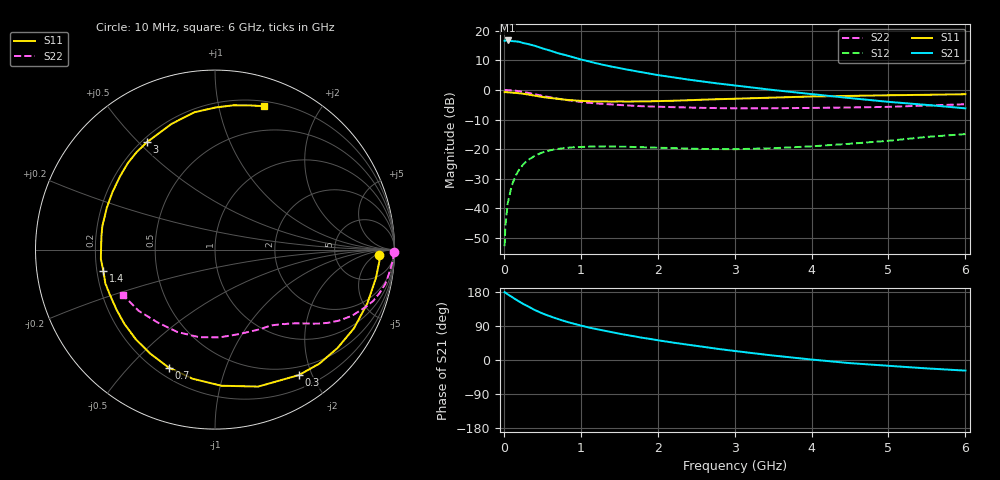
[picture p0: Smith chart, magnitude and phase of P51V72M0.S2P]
! SIEMENS Small Signal Semiconductors
! BFP183
! Si NPN RF Bipolar Junction Transistor in SOT143
! VCE = 1.75 V  IC = 2 mA
! Common Emitter S-Parameters:  March  1996
# GHz  S  MA  R  50
!  f  S11  S21  S12  S22
! GHz  MAG  ANG  MAG  ANG  MAG  ANG  MAG  ANG
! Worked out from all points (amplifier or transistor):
!   36 points, 10 MHz to 6 GHz, reference 50 ohm
!   highest |S21| = 16.7 dB at 50 MHz (marker M1)
!   |S21| within 3 dB of that: start of sweep to 545.6 MHz
!   unconditionally stable (mu >= 1): 2.063 GHz to end of sweep
!   at 250 MHz: K = 0.12, MSG = 20.5 dB, |S12| = -25.2 dB
!   at 1.4 GHz: K = 0.68, MSG = 13.5 dB, |S12| = -19.1 dB
!   at 6 GHz: K = 1.01, MAG = 3.8 dB, |S12| = -14.9 dB
!   S11 on the Smith chart (normalised r, x): 10 MHz: 20, -7; 300 MHz: 0.38, -1.81; 700 MHz: 0.25, -0.65; 1.4 GHz: 0.23, -0.09; 3 GHz: 0.22, +0.53; 6 GHz: 0.25, +1.37
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0.01  0.9157 -1.9  6.767 179.0  0.0023 85.0  0.9985 -0.7
0.02  0.9182 -4.0  6.789 177.9  0.005 85.8  0.9963 -1.6
0.05  0.9106 -10.0  6.829 173.4  0.0121 86.4  0.9915 -3.8
0.1  0.9001 -19.4  6.672 167.0  0.0236 78.7  0.9797 -7.6
0.2  0.8755 -38.8  6.478 154.1  0.0453 68.5  0.9488 -14.7
0.25  0.8614 -47.5  6.182 148.3  0.0547 63.4  0.9267 -18.0
0.3  0.8411 -56.2  6.004 143.1  0.0634 59.1  0.8996 -20.7
0.4  0.8002 -72.5  5.562 132.1  0.077 50.8  0.8474 -25.8
0.5  0.7593 -87.3  5.032 123.0  0.0878 43.5  0.7947 -29.9
0.6  0.7304 -99.7  4.609 115.4  0.0955 37.9  0.7509 -32.9
0.7  0.706 -111.5  4.17 108.4  0.1009 32.8  0.7116 -35.4
0.8  0.6824 -122.0  3.867 101.9  0.1043 28.9  0.6791 -37.4
0.9  0.6664 -131.5  3.561 96.3  0.1076 25.3  0.6496 -39.3
1.1  0.6428 -148.6  3.04 86.0  0.1101 19.7  0.6065 -42.6
1.4  0.6332 -169.3  2.471 73.6  0.1111 13.7  0.5685 -46.9
1.8  0.6412 168.2  1.982 58.7  0.1076 10.3  0.5299 -52.6
2.2  0.6554 150.4  1.63 45.9  0.1042 8.5  0.5115 -59.3
3  0.7086 122.3  1.189 23.8  0.0996 12.1  0.4884 -75.3
3.5  0.7408 109.1  0.996 11.8  0.1036 16.4  0.4895 -86.7
4.5  0.792 89.7  0.727 -8.3  0.1233 22.2  0.5047 -114.6
5.5  0.8265 76.4  0.557 -22.2  0.1608 22.3  0.5454 -141.3
6  0.8448 71.0  0.488 -28.0  0.1794 18.9  0.572 -153.9
